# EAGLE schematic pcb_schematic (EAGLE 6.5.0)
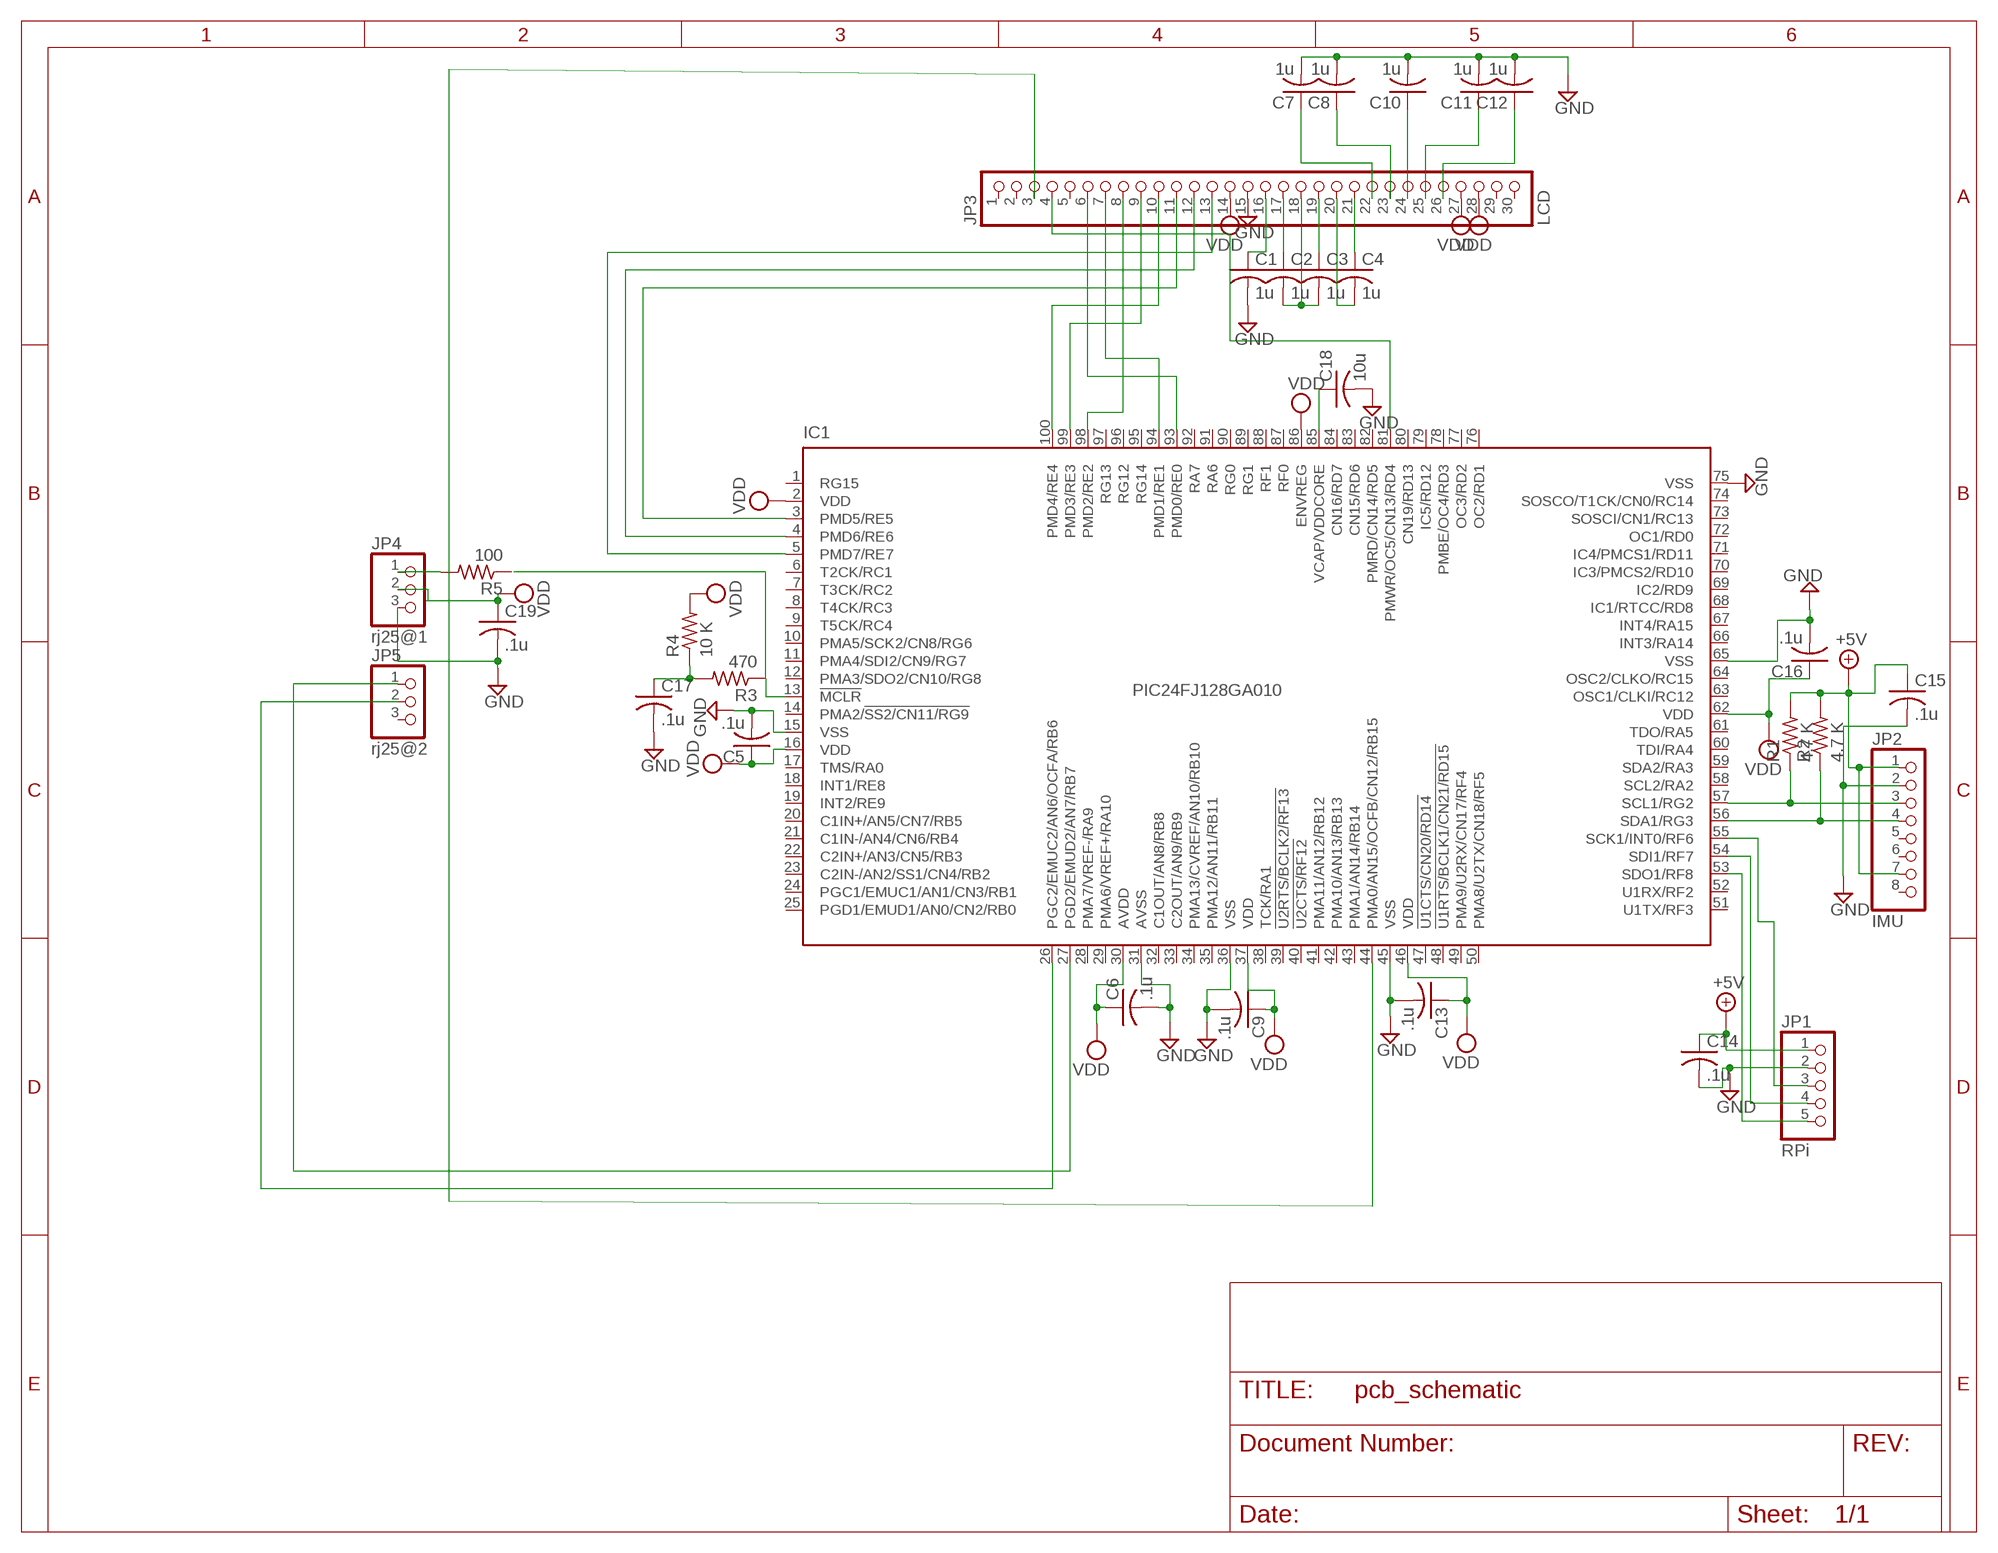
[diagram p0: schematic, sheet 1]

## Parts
C1  1u  C-USC1206K  [C1206K]
C2  1u  C-USC1206K  [C1206K]
C3  1u  C-USC1206K  [C1206K]
C4  1u  C-USC1206K  [C1206K]
C5  .1u  C-USC1206K  [C1206K]
C6  .1u  C-USC1206K  [C1206K]
C7  1u  C-USC1206K  [C1206K]
C8  1u  C-USC1206K  [C1206K]
C9  .1u  C-USC1206K  [C1206K]
C10  1u  C-USC1206K  [C1206K]
C11  1u  C-USC1206K  [C1206K]
C12  1u  C-USC1206K  [C1206K]
C13  .1u  C-USC1206K  [C1206K]
C14  .1u  C-USC1206K  [C1206K]
C15  .1u  C-USC1206K  [C1206K]
C16  .1u  C-USC1206K  [C1206K]
C17  .1u  C-USC1206K  [C1206K]
C18  10u  C-USC1206K  [C1206K]
C19  .1u  C-USC1206K  [C1206K]
IC1  PIC24FJ128GA010  [TQFP100-14X14]
JP1  RPi  PINHD-1X5  [1X05]
JP2  IMU  PINHD-1X8  [1X08]
JP3  LCD  PINHD-1X30  [1X30]
JP4  rj25@1  PINHD-1X3  [1X03]
JP5  rj25@2  PINHD-1X3  [1X03]
R1  4.7 K  R-US_M2012  [M2012]
R2  4.7 K  R-US_M2012  [M2012]
R3  470  R-US_M2012  [M2012]
R4  10 K  R-US_M2012  [M2012]
R5  100  R-US_M2012  [M2012]

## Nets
+5V: C14.1 C15.1 JP1.1 JP2.1 JP2.7 R1.2 R2.2
GND: C1.2 C5.2 C6.2 C7.2 C8.2 C9.2 C10.2 C11.2 C12.2 C13.2 C14.2 C15.2 C16.2 C17.2 C18.2 C19.2 IC1.15(VSS) IC1.31(AVSS) IC1.36(VSS) IC1.45(VSS) IC1.65(VSS) IC1.75(VSS) JP1.2 JP2.2 JP3.15 JP4.3
N$1: IC1.57(SCL1/RG2) JP2.3 R1.1
N$2: IC1.56(SDA1/RG3) JP2.4 R2.1
N$3: IC1.44(PMA0/AN15/OCFB/CN12/RB15) JP3.3
N$4: IC1.55(SCK1/INT0/RF6) JP1.3
N$5: IC1.54(SDI1/RF7) JP1.4
N$6: IC1.53(SDO1/RF8) JP1.5
N$7: C18.1 IC1.85(VCAP/VDDCORE)
N$8: IC1.5(PMD7/RE7) JP3.13
N$9: IC1.4(PMD6/RE6) JP3.12
N$10: IC1.3(PMD5/RE5) JP3.11
N$11: IC1.100(PMD4/RE4) JP3.10
N$12: IC1.99(PMD3/RE3) JP3.9
N$13: IC1.98(PMD2/RE2) JP3.8
N$14: IC1.94(PMD1/RE1) JP3.7
N$15: IC1.93(PMD0/RE0) JP3.6
N$16: C7.1 JP3.22
N$17: C3.1 JP3.19
N$18: IC1.81(PMWR/OC5/CN13/RD4) JP3.4
N$19: C2.1 JP3.17
N$20: C2.2 C3.2 JP3.18
N$21: C1.1 JP3.16
N$22: C4.2 JP3.20
N$23: C4.1 JP3.21
N$24: C8.1 JP3.23
N$25: C10.1 JP3.24
N$26: C11.1 JP3.25
N$27: C12.1 JP3.26
N$28: IC1.13(!MCLR) R3.1
N$29: JP4.1 R5.2
N$30: C17.1 R3.2 R4.1
N$31: JP4.2
N$32: IC1.26(PGC2/EMUC2/AN6/OCFA/RB6) JP5.2
N$33: IC1.27(PGD2/EMUD2/AN7/RB7) JP5.1
VDD: C5.1 C6.1 C9.1 C13.1 C16.1 C19.1 IC1.2(VDD) IC1.16(VDD) IC1.30(AVDD) IC1.37(VDD) IC1.46(VDD) IC1.62(VDD) IC1.86(ENVREG) JP3.14 JP3.27 JP3.28 R4.2
Unconnected: IC1.1(RG15) IC1.6(T2CK/RC1) IC1.7(T3CK/RC2) IC1.8(T4CK/RC3) IC1.9(T5CK/RC4) IC1.10(PMA5/SCK2/CN8/RG6) IC1.11(PMA4/SDI2/CN9/RG7) IC1.12(PMA3/SDO2/CN10/RG8) IC1.14(PMA2/!SS2/CN11/RG9) IC1.17(TMS/RA0) IC1.18(INT1/RE8) IC1.19(INT2/RE9) IC1.20(C1IN+/AN5/CN7/RB5) IC1.21(C1IN-/AN4/CN6/RB4) IC1.22(C2IN+/AN3/CN5/RB3) IC1.23(C2IN-/AN2/SS1/CN4/RB2) IC1.24(PGC1/EMUC1/AN1/CN3/RB1) IC1.25(PGD1/EMUD1/AN0/CN2/RB0) IC1.28(PMA7/VREF-/RA9) IC1.29(PMA6/VREF+/RA10) IC1.32(C1OUT/AN8/RB8) IC1.33(C2OUT/AN9/RB9) IC1.34(PMA13/CVREF/AN10/RB10) IC1.35(PMA12/AN11/RB11) IC1.38(TCK/RA1) IC1.39(!U2RTS/BCLK2/RF13) IC1.40(!U2CTS/RF12) IC1.41(PMA11/AN12/RB12) IC1.42(PMA10/AN13/RB13) IC1.43(PMA1/AN14/RB14) IC1.47(!U1CTS/CN20/RD14) IC1.48(!U1RTS/BCLK1/CN21/RD15) IC1.49(PMA9/U2RX/CN17/RF4) IC1.50(PMA8/U2TX/CN18/RF5) IC1.51(U1TX/RF3) IC1.52(U1RX/RF2) IC1.58(SCL2/RA2) IC1.59(SDA2/RA3) IC1.60(TDI/RA4) IC1.61(TDO/RA5) IC1.63(OSC1/CLKI/RC12) IC1.64(OSC2/CLKO/RC15) IC1.66(INT3/RA14) IC1.67(INT4/RA15) IC1.68(IC1/RTCC/RD8) IC1.69(IC2/RD9) IC1.70(IC3/PMCS2/RD10) IC1.71(IC4/PMCS1/RD11) IC1.72(OC1/RD0) IC1.73(SOSCI/CN1/RC13) IC1.74(SOSCO/T1CK/CN0/RC14) IC1.76(OC2/RD1) IC1.77(OC3/RD2) IC1.78(PMBE/OC4/RD3) IC1.79(IC5/RD12) IC1.80(CN19/RD13) IC1.82(PMRD/CN14/RD5) IC1.83(CN15/RD6) IC1.84(CN16/RD7) IC1.87(RF0) IC1.88(RF1) IC1.89(RG1) IC1.90(RG0) IC1.91(RA6) IC1.92(RA7) IC1.95(RG14) IC1.96(RG12) IC1.97(RG13) JP2.5 JP2.6 JP2.8 JP3.1 JP3.2 JP3.5 JP3.29 JP3.30 JP5.3 R5.1

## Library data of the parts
C1-C19 = rcl:C-US: CAPACITOR, American symbol
IC1 = microchip:PIC24FJ*GA010: 64/80/100-Pin General Purpose, 16-Bit Flash Microcontrollers Source: http://ww1.microchip.com/downloads/en/DeviceDoc/39747d.pdf; MPN: PIC24FJ128GA010-I/PT; OC_FARNELL: 1146522; OC_NEWARK: 56K7341
JP1 = pinhead:PINHD-1X5: PIN HEADER
JP2 = pinhead:PINHD-1X8: PIN HEADER
JP3 = pinhead:PINHD-1X30: PIN HEADER
JP4 JP5 = pinhead:PINHD-1X3: PIN HEADER
R1-R5 = rcl:R-US_: RESISTOR, American symbol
